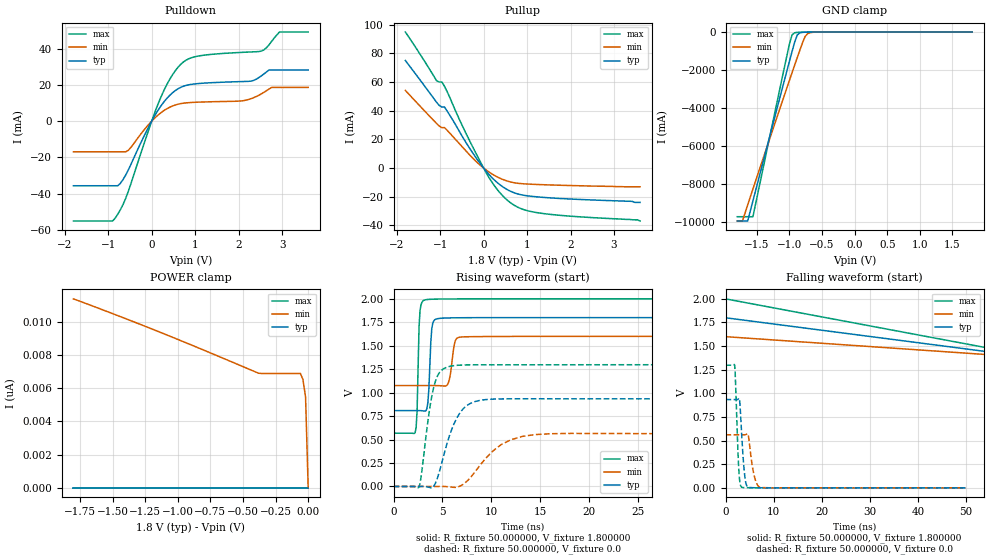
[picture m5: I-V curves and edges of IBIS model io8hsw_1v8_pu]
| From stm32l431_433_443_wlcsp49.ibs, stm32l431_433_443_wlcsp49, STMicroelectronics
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|   Model io8hsw_1v8_pu
[Model]  io8hsw_1v8_pu
Model_type I/O
Polarity   Non-Inverting
Enable   Active-Low
Vinl =   0.540000V
Vinh =   1.260000V
Vmeas =  0.900000V
Cref =   100.000000nF
Rref =   1.000000k
Vref =   1.800000V
C_comp   3.002500pF   2.845500pF   3.023700pF
[Temperature Range]   25.000000   0.125000k   -40.000000
[Pullup Reference]   1.800000V   1.600000V   2.000000V
[Pulldown Reference]   0.0V   0.0V   0.0V
[POWER Clamp Reference]   1.800000V   1.600000V   2.000000V
[GND Clamp Reference]   0.0V   0.0V   0.0V
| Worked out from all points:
|   slope of the pulldown table from 0 to 0.27 V, typ, clamps not added: 26.4 ohm
|   slope of the pullup table from 0 to 0.27 V, typ, clamps not added: 30.1 ohm
|   GND clamp passes 1 mA (typ) near -0.58 V on its own axis
|   rising waveform, R_fixture 50.000000, V_fixture 1.800000: 20-80 % time 264ps typ, 405ps min, 197ps max; typ from 0.809 V to 1.8 V
|   rising waveform, R_fixture 50.000000, V_fixture 0.0: 20-80 % time 1.8ns typ, 3.06ns min, 1.06ns max; typ from 0 V to 0.934 V
|   falling waveform, R_fixture 50.000000, V_fixture 1.800000: 20-80 % time 90.1ns typ, 90.1ns min, 90.1ns max; typ from 1.8 V to 0.809 V
|   falling waveform, R_fixture 50.000000, V_fixture 0.0: 20-80 % time 718ps typ, 1.03ns min, 555ps max; typ from 0.934 V to 0 V
[Pulldown]
|Voltage   I(typ)   I(min)   I(max)
-1.8V     -35.64mA   -16.93mA   -55.1mA
-840mV    -35.64mA   -16.93mA   -53.52mA
-720mV    -34.31mA   -16.93mA   -48.86mA
-540mV    -27.04mA   -16.13mA   -38.89mA
240mV     9.303mA    5.14mA     14.78mA
480mV     15.67mA    8.374mA    25.64mA
720mV     19.18mA    9.883mA    32.46mA
1.08V     20.76mA    10.49mA    35.96mA
2.1V      21.86mA    11.27mA    37.98mA
2.52V     24.96mA    15.02mA    38.63mA
2.94V     28.26mA    18.61mA    49.17mA
3.6V      28.26mA    18.61mA    49.17mA
[Pullup]
|Voltage   I(typ)   I(min)   I(max)
-1.8V     75.07mA    54.19mA    94.94mA
-1.08V    45.8mA     31.06mA    60.87mA
-960mV    42.59mA    28.22mA    60.05mA
-900mV    42.58mA    28.22mA    57.06mA
-480mV    21.53mA    14.44mA    28.9mA
-240mV    10.08mA    6.588mA    14.1mA
0V        40fA       13.9pA     0A
300mV     -9.801mA   -6.008mA   -14.46mA
600mV     -15.96mA   -9.582mA   -23.81mA
900mV     -18.89mA   -10.98mA   -28.81mA
1.32V     -20.37mA   -11.6mA    -31.56mA
3.6V      -24mA      -13.1mA    -37mA
[GND_clamp]
|Voltage   I(typ)   I(min)   I(max)
-1.8V     -9.93A     -9.932A    -9.707A
-1.72V    -9.93A     -9.932A    -9.707A
-1.64V    -9.93A     -9.083A    -9.707A
-1.56V    -8.876A    -8.251A    -9.707A
-1V       -1.54A     -2.541A    -631mA
-960mV    -1.028A    -2.139A    -153.7mA
-920mV    -527mA     -1.74A     -39.12mA
-880mV    -155.6mA   -1.344A    -18.01mA
-840mV    -45.32mA   -953mA     -12.68mA
-760mV    -8.418mA   -235mA     -7.62mA
-680mV    -3.44mA    -33.01mA   -3.865mA
1.8V      0A         0A         0A
[POWER_clamp]
|Voltage   I(typ)   I(min)   I(max)
-1.8V     0A         11.37nA    0A
-1.14V    0A         9.374nA    0A
-380mV    0A         6.895nA    0A
-60mV     0A         6.881nA    0A
-40mV     0A         6.518nA    0A
-20mV     0A         5.452nA    0A
0V        0A         0A         0A
[Ramp]
| variable   typ   min   max
dV/dt_r  0.56063/1.80220n   0.33686/3.05671n   0.77868/1.05812n
dV/dt_f  0.59464/1.73024n   0.31464/3.04463n   0.85906/0.96420n
R_load = 50.000000
[Rising Waveform]
R_fixture= 50.000000
V_fixture= 1.800000
V_fixture_min= 1.600000
V_fixture_max= 2.000000
|time   V(typ)   V(min)   V(max)
0s        808.7mV    1.076V     568.2mV
2.202ns   808.8mV    1.076V     574.9mV
2.402ns   808.8mV    1.076V     804mV
2.703ns   808.5mV    1.076V     1.874V
3.203ns   802.9mV    1.076V     1.989V
3.504ns   892.4mV    1.076V     1.994V
3.904ns   1.68V      1.076V     1.996V
4.505ns   1.789V     1.075V     1.998V
6.907ns   1.799V     1.593V     2V
49.85ns   1.8V       1.6V       2V
[Rising Waveform]
R_fixture= 50.000000
V_fixture= 0.0
V_fixture_min= 0.0
V_fixture_max= 0.0
|time   V(typ)   V(min)   V(max)
0s        2.998nV    80.83nV    2.225nV
2.603ns   15.19uV    -22.24nV   -7.666mV
3.704ns   -11.07mV   680.5pV    838mV
4.204ns   19.29mV    9.234uV    1.096V
5.906ns   595.3mV    -6.329mV   1.284V
6.807ns   788mV      4.452mV    1.294V
8.108ns   896.9mV    125.8mV    1.296V
11.01ns   933.4mV    446.5mV    1.297V
14.41ns   934.8mV    552.1mV    1.297V
49.85ns   934.4mV    561.5mV    1.298V
[Falling Waveform]
R_fixture= 50.000000
V_fixture= 1.800000
V_fixture_min= 1.600000
V_fixture_max= 2.000000
|time   V(typ)   V(min)   V(max)
0s        1.8V       1.6V       2V
150.2ns   808.8mV    1.076V     568.2mV
1.051us   808.7mV    1.076V     568.2mV
14.86us   808.7mV    1.076V     568.2mV
[Falling Waveform]
R_fixture= 50.000000
V_fixture= 0.0
V_fixture_min= 0.0
V_fixture_max= 0.0
|time   V(typ)   V(min)   V(max)
0s        934.4mV    561.5mV    1.298V
1.902ns   934.4mV    561.5mV    1.3V
2.803ns   948mV      561.5mV    156.9mV
3.403ns   522mV      561.4mV    5.865mV
3.904ns   172mV      561.1mV    2.319mV
4.304ns   36.57mV    566.3mV    1.568mV
4.705ns   8.397mV    560.8mV    1.191mV
5.906ns   1.314mV    138.6mV    625uV
7.207ns   549.6uV    5.718mV    408.3uV
49.85ns   2.998nV    80.83nV    2.225nV
